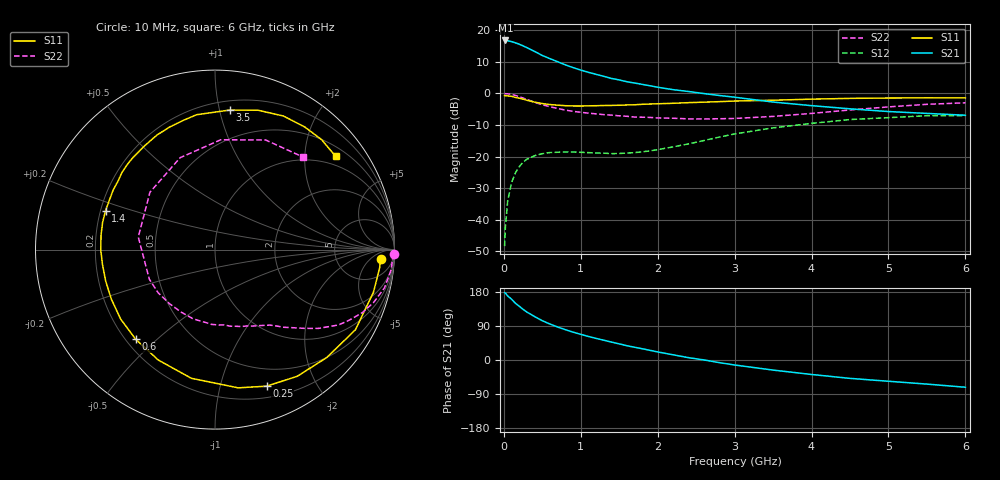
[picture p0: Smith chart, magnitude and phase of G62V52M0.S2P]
! SIEMENS Small Signal Semiconductors
! BFG193
! Si NPN RF Bipolar Junction Transistor in SOT223
! VCE = 2.5 V  IC = 2 mA
! Common Emitter S-Parameters:  August  1996
# GHz  S  MA  R  50
!  f  S11  S21  S12  S22
! GHz  MAG  ANG  MAG  ANG  MAG  ANG  MAG  ANG
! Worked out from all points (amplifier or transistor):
!   36 points, 10 MHz to 6 GHz, reference 50 ohm
!   highest |S21| = 16.8 dB at 20 MHz (marker M1)
!   |S21| within 3 dB of that: start of sweep to 360 MHz
!   unconditionally stable (mu >= 1): 1.37 GHz to 2.646 GHz
!   at 250 MHz: K = 0.18, MSG = 18.4 dB, |S12| = -21.8 dB
!   at 1.4 GHz: K = 1.03, MAG = 10.9 dB, |S12| = -19.1 dB
!   at 6 GHz: K = 0.97, MSG = 0.1 dB, |S12| = -7.0 dB
!   S11 on the Smith chart (normalised r, x): 10 MHz: 17, -12; 250 MHz: 0.31, -1.40; 600 MHz: 0.24, -0.43; 1.4 GHz: 0.22, +0.16; 3.5 GHz: 0.27, +1.07; 6 GHz: 0.74, +2.75
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0.01  0.9244 -3.2  6.833 177.8  0.0038 93.8  0.9964 -1.4
0.02  0.9229 -6.3  6.921 176.6  0.0075 84.0  0.9907 -2.6
0.05  0.9142 -15.1  6.852 169.0  0.0199 80.9  0.9881 -6.5
0.1  0.9009 -29.7  6.644 160.5  0.0384 74.4  0.9682 -12.7
0.15  0.8656 -44.0  6.348 149.8  0.0551 65.4  0.9317 -18.4
0.2  0.8415 -57.0  6.042 142.0  0.069 59.0  0.8925 -23.2
0.25  0.8133 -69.3  5.685 133.7  0.0814 52.5  0.8454 -27.7
0.3  0.7809 -80.5  5.322 126.5  0.0907 47.4  0.8061 -31.4
0.4  0.729 -100.4  4.637 114.6  0.1032 38.4  0.7244 -37.3
0.5  0.6917 -117.2  4.003 103.6  0.111 31.7  0.6621 -41.5
0.6  0.6669 -131.5  3.559 94.9  0.1159 27.0  0.6155 -45.0
0.7  0.6527 -143.7  3.18 87.0  0.1171 23.1  0.5777 -48.5
0.8  0.6401 -154.4  2.838 80.0  0.1183 20.2  0.545 -51.3
1.1  0.6365 -179.8  2.162 62.1  0.1154 16.5  0.4873 -60.5
1.4  0.6472 160.4  1.729 47.2  0.1113 17.4  0.4534 -70.9
1.7  0.6613 144.8  1.463 33.6  0.1154 23.3  0.4227 -83.0
2.2  0.6986 124.2  1.149 13.7  0.1424 29.6  0.4048 -107.3
2.8  0.7416 103.7  0.93 -6.9  0.2035 27.9  0.3976 -142.9
3.5  0.7818 84.0  0.731 -26.6  0.285 13.7  0.4331 170.7
4.5  0.8361 62.9  0.571 -48.5  0.3862 -10.1  0.5476 110.8
5.5  0.8532 45.9  0.483 -63.6  0.4439 -38.3  0.6728 65.2
6  0.8497 37.7  0.452 -71.9  0.4445 -53.4  0.7117 46.4
